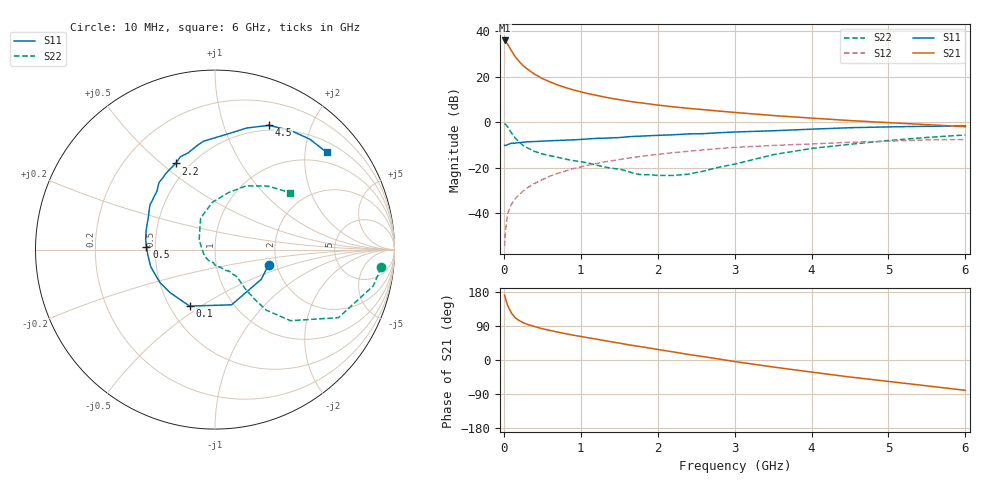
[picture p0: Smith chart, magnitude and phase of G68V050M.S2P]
! SIEMENS Small Signal Semiconductors
! BFG193
! Si NPN RF Bipolar Junction Transistor in SOT223
! VCE = 8 V  IC = 50 mA
! Common Emitter S-Parameters:  August  1996
# GHz  S  MA  R  50
!  f  S11  S21  S12  S22
! GHz  MAG  ANG  MAG  ANG  MAG  ANG  MAG  ANG
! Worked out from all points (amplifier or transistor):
!   36 points, 10 MHz to 6 GHz, reference 50 ohm
!   highest |S21| = 35.8 dB at 10 MHz (marker M1)
!   |S21| within 3 dB of that: start of sweep to 72.8 MHz
!   unconditionally stable (mu >= 1): 487.6 MHz to 2.38 GHz
!   at 250 MHz: K = 0.89, MSG = 27.5 dB, |S12| = -30.3 dB
!   at 1.4 GHz: K = 1.04, MAG = 12.4 dB, |S12| = -17.0 dB
!   at 6 GHz: K = 0.89, MSG = 2.8 dB, |S12| = -7.6 dB
!   S11 on the Smith chart (normalised r, x): 10 MHz: 1.81, -0.34; 100 MHz: 0.63, -0.45; 500 MHz: 0.45, +0.02; 2.2 GHz: 0.42, +0.56; 4.5 GHz: 0.44, +1.43; 6 GHz: 0.73, +2.49
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0.01  0.3105 -15.9  61.92 171.0  0.0019 94.1  0.9313 -6.1
0.02  0.3063 -32.7  59.7 163.7  0.004 79.1  0.9049 -12.9
0.05  0.3212 -73.3  50.96 143.3  0.0099 72.0  0.785 -28.9
0.1  0.3451 -114.2  36.63 123.5  0.016 67.9  0.5774 -43.3
0.15  0.3468 -136.4  26.98 111.0  0.021 65.8  0.4425 -49.7
0.2  0.3568 -148.9  21.35 104.1  0.0257 66.3  0.3652 -51.2
0.25  0.3613 -157.7  17.45 98.5  0.0307 67.6  0.3085 -51.9
0.3  0.3707 -165.1  14.79 94.4  0.0357 68.2  0.2759 -52.3
0.4  0.3746 -174.5  11.27 88.3  0.0453 68.8  0.228 -51.7
0.5  0.3828 177.5  9.059 82.6  0.0548 68.1  0.2004 -51.1
0.6  0.3902 171.6  7.611 78.0  0.0654 67.2  0.1836 -52.0
0.7  0.3959 166.3  6.554 73.6  0.0749 65.9  0.1692 -54.0
0.8  0.402 161.3  5.734 69.5  0.0847 64.0  0.1544 -55.5
1.1  0.4285 148.8  4.204 58.6  0.1138 59.1  0.126 -64.9
1.3  0.4436 142.0  3.574 51.5  0.1334 55.1  0.1046 -71.9
1.6  0.4758 131.8  2.913 40.9  0.1607 48.3  0.0846 -91.0
2.2  0.5276 114.6  2.167 21.4  0.2135 34.9  0.0676 -152.3
2.8  0.5854 100.3  1.745 2.4  0.2636 21.0  0.1033 148.9
3.5  0.6463 84.1  1.397 -18.5  0.3084 3.9  0.1932 114.5
4.5  0.7543 66.6  1.082 -44.9  0.3624 -16.1  0.3263 76.7
5.5  0.8107 49.4  0.881 -68.2  0.4085 -39.2  0.4614 50.1
6  0.8255 41.0  0.793 -80.1  0.4149 -52.6  0.5236 37.4
